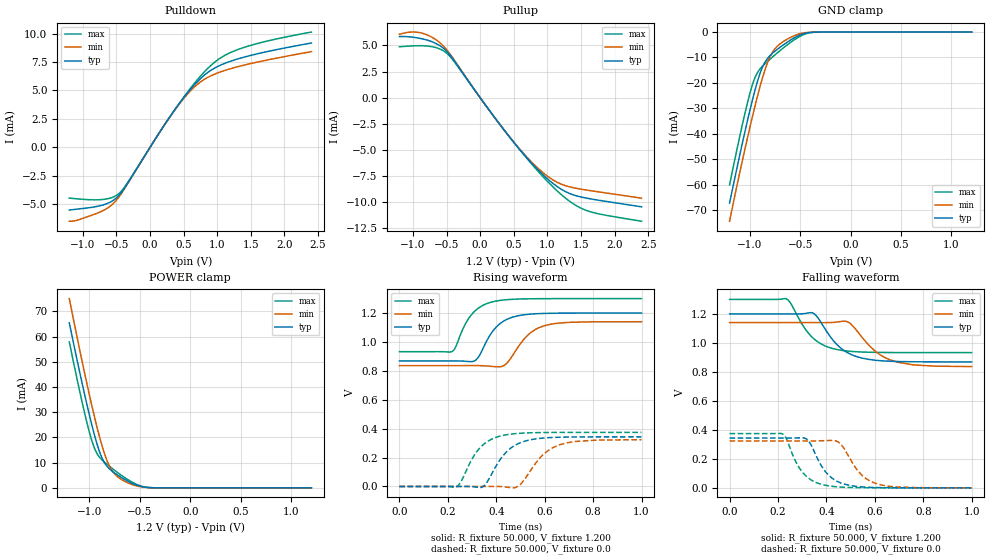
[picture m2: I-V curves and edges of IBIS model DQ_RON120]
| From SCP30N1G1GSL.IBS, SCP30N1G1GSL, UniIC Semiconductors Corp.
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|   Model DQ_RON120
[Model] DQ_RON120
Model_type I/O
Vinl =  0.500V
Vinh =  0.700V
Vmeas =  0.600V
Rref =  50.000
Vref =  0.600V
C_comp   1.373pF   1.353pF   1.403pF
[Model Spec]
Vinh   0.700V   0.670V   0.750V
Vinl   0.500V   0.470V   0.550V
Vmeas   0.600V   0.570V   0.650V
Vref   0.600V   0.570V   0.650V
Rref   50.000   NA   NA
[Temperature Range]   25.000   85.000   -40.000
[Voltage Range]   1.200V   1.140V   1.300V
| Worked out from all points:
|   slope of the pulldown table from 0 to 0.18 V, typ, clamps not added: 108 ohm
|   slope of the pullup table from 0 to 0.18 V, typ, clamps not added: 113 ohm
|   GND clamp passes 1 mA (typ) near -0.49 V on its own axis
|   POWER clamp passes 1 mA (typ) near -0.53 V on its own axis
|   rising waveform, R_fixture 50.000, V_fixture 1.200: 20-80 % time 81.6ps typ, 91.9ps min, 78.4ps max; typ from 0.869 V to 1.2 V
|   rising waveform, R_fixture 50.000, V_fixture 0.0: 20-80 % time 92.5ps typ, 101ps min, 87.1ps max; typ from 0 V to 0.343 V
|   falling waveform, R_fixture 50.000, V_fixture 1.200: 20-80 % time 104ps typ, 116ps min, 97.4ps max; typ from 1.2 V to 0.869 V
|   falling waveform, R_fixture 50.000, V_fixture 0.0: 20-80 % time 79.1ps typ, 85.5ps min, 75.9ps max; typ from 0.343 V to 0 V
[Pulldown]
|Voltage   I(typ)   I(min)   I(max)
-1.2V     -5.501mA   -6.484mA   -4.453mA
-719mV    -5.085mA   -5.607mA   -4.58mA
-571mV    -4.739mA   -5.06mA    -4.412mA
-460mV    -4.203mA   -4.337mA   -4.038mA
-349mV    -3.3mA     -3.343mA   -3.237mA
317mV     2.872mA    2.858mA    2.868mA
576mV     4.923mA    4.804mA    4.997mA
761mV     6.104mA    5.797mA    6.33mA
1.02V     7.148mA    6.572mA    7.743mA
1.279V    7.725mA    7.046mA    8.535mA
1.723V    8.39mA     7.653mA    9.313mA
2.4V      9.17mA     8.411mA    10.13mA
[Pullup]
|Voltage   I(typ)   I(min)   I(max)
-1.2V     5.842mA    6.067mA    4.866mA
-1.004V   5.781mA    6.272mA    4.949mA
-819mV    5.558mA    6.073mA    4.949mA
-634mV    5.104mA    5.434mA    4.739mA
-486mV    4.358mA    4.495mA    4.193mA
69mV      -617.5uA   -621.6uA   -608.7uA
439mV     -3.773mA   -3.764mA   -3.761mA
772mV     -6.298mA   -6.197mA   -6.381mA
1.031V    -7.923mA   -7.641mA   -8.198mA
1.29V     -9.043mA   -8.453mA   -9.702mA
1.549V    -9.561mA   -8.796mA   -10.7mA
2.4V      -10.43mA   -9.609mA   -11.81mA
[GND_clamp]
|Voltage   I(typ)   I(min)   I(max)
-1.2V     -67.26mA   -74.42mA   -60.1mA
-1.05V    -39.62mA   -46.47mA   -32.4mA
-1V       -31.05mA   -37.77mA   -24.37mA
-950mV    -23.16mA   -29.46mA   -18.1mA
-925mV    -19.62mA   -25.5mA    -16.02mA
-875mV    -13.89mA   -18.21mA   -13.48mA
-825mV    -10.4mA    -12.16mA   -11.61mA
-775mV    -8.365mA   -7.964mA   -9.852mA
-700mV    -6.001mA   -4.671mA   -7.319mA
-525mV    -1.587mA   -933.3uA   -2.208mA
-375mV    -90.13uA   -49.22uA   -132.9uA
1.2V      0A         0A         0A
[POWER_clamp]
|Voltage   I(typ)   I(min)   I(max)
-1.2V     65.51mA    75.11mA    57.91mA
-1.05V    37.38mA    45.87mA    29.99mA
-1V       28.74mA    36.73mA    21.95mA
-950mV    20.85mA    28.08mA    15.65mA
-925mV    17.34mA    24.01mA    13.56mA
-875mV    11.74mA    16.61mA    11.06mA
-825mV    8.457mA    10.65mA    9.317mA
-775mV    6.603mA    6.7mA      7.708mA
-725mV    5.177mA    4.492mA    6.178mA
-550mV    1.336mA    943.1uA    1.707mA
-400mV    85.95uA    67.55uA    91.19uA
1.2V      0A         0A         0A
[Ramp]
| variable   typ   min   max
dV/dt_r   0.206/92.488p   0.194/0.100n   0.225/87.374p
dV/dt_f   0.199/0.105n   0.182/0.116n   0.220/97.570p
R_load = 50.000
[Rising Waveform]
R_fixture= 50.000
V_fixture= 1.200
V_fixture_min= 1.140
V_fixture_max= 1.300
|time   V(typ)   V(min)   V(max)
0s        868.7mV    836.1mV    932.8mV
218ps     869mV      836mV      934.3mV
278ps     865.5mV    836.4mV    1.142V
316ps     875.2mV    836.5mV    1.221V
390ps     1.084V     829.6mV    1.28V
436ps     1.149V     841.6mV    1.291V
517ps     1.189V     1.024V     1.298V
593ps     1.197V     1.109V     1.3V
704ps     1.2V       1.136V     1.3V
1ns       1.2V       1.14V      1.3V
[Rising Waveform]
R_fixture= 50.000
V_fixture= 0.0
V_fixture_min= 0.0
V_fixture_max= 0.0
|time   V(typ)   V(min)   V(max)
0s        62.39nV    201nV      36.07nV
236ps     66.72uV    -5.383uV   -1.609mV
254ps     251.9uV    -17.76uV   32.91mV
303ps     -1.391mV   -15.78uV   199.2mV
342ps     -4.396mV   183.3uV    283.1mV
423ps     202.2mV    -1.267mV   351.7mV
492ps     297.4mV    3.79mV     367.4mV
593ps     334.9mV    219.3mV    373.2mV
663ps     340.8mV    289.2mV    374mV
1ns       343.4mV    323.7mV    374.4mV
[Falling Waveform]
R_fixture= 50.000
V_fixture= 1.200
V_fixture_min= 1.140
V_fixture_max= 1.300
|time   V(typ)   V(min)   V(max)
0s        1.2V       1.14V      1.3V
233ps     1.2V       1.14V      1.305V
314ps     1.203V     1.14V      1.092V
351ps     1.2V       1.14V      1.024V
442ps     991mV      1.143V     954.7mV
493ps     927.3mV    1.141V     942.7mV
602ps     880.2mV    942mV      934.6mV
662ps     873.3mV    883.6mV    933.5mV
760ps     869.7mV    848.1mV    933mV
1ns       868.7mV    836.5mV    932.9mV
[Falling Waveform]
R_fixture= 50.000
V_fixture= 0.0
V_fixture_min= 0.0
V_fixture_max= 0.0
|time   V(typ)   V(min)   V(max)
0s        343.5mV    323.9mV    374.4mV
221ps     343.3mV    323.9mV    369.9mV
282ps     344.5mV    323.8mV    153.9mV
321ps     333.3mV    323.6mV    73.84mV
388ps     129.3mV    325.2mV    20.63mV
455ps     36.95mV    308.1mV    5.754mV
530ps     8.902mV    117mV      1.39mV
601ps     2.341mV    31.9mV     357.3uV
690ps     431.5uV    6.051mV    65.33uV
1ns       1.245uV    17.74uV    209.4nV
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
